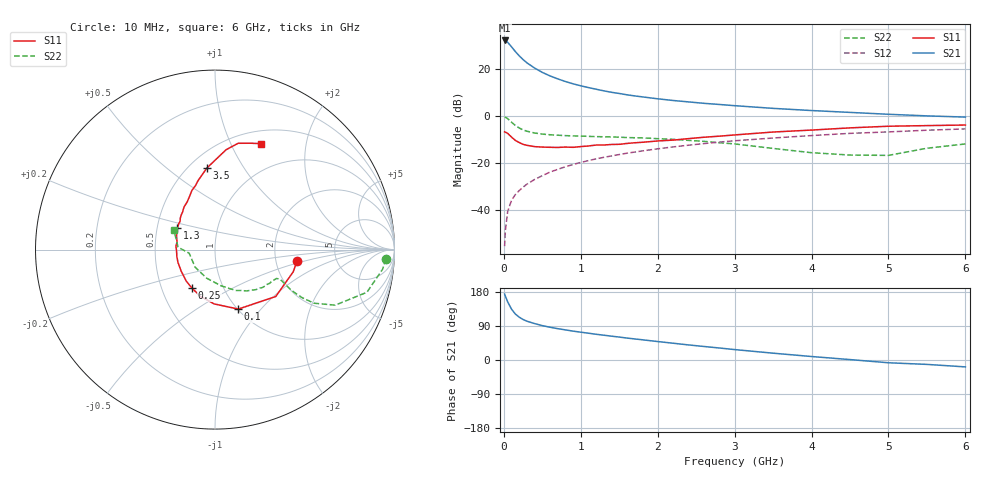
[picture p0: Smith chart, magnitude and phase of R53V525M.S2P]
! SIEMENS Small Signal Semiconductors
! BFR183
! Si NPN RF Bipolar Junction Transistor in SOT23
! VCE = 3.5 V  IC = 25 mA
! Common Emitter S-Parameters:  May  1996
# GHz  S  MA  R  50
!  f  S11  S21  S12  S22
! GHz  MAG  ANG  MAG  ANG  MAG  ANG  MAG  ANG
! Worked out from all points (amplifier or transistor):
!   36 points, 10 MHz to 6 GHz, reference 50 ohm
!   highest |S21| = 32.2 dB at 10 MHz (marker M1)
!   |S21| within 3 dB of that: start of sweep to 107.2 MHz
!   unconditionally stable (mu >= 1): 483.5 MHz to 2.364 GHz
!   at 250 MHz: K = 0.86, MSG = 27.2 dB, |S12| = -30.3 dB
!   at 1.4 GHz: K = 1.04, MAG = 12.3 dB, |S12| = -17.0 dB
!   at 6 GHz: K = 0.90, MSG = 2.5 dB, |S12| = -5.5 dB
!   S11 on the Smith chart (normalised r, x): 10 MHz: 2.63, -0.43; 100 MHz: 1.01, -0.76; 250 MHz: 0.71, -0.32; 1.3 GHz: 0.64, +0.16; 3.5 GHz: 0.61, +0.70; 6 GHz: 0.65, +1.31
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0.01  0.4613 -8.1  40.55 174.0  0.0017 85.6  0.9526 -3.1
0.02  0.4529 -15.9  39.98 168.4  0.0037 85.2  0.9402 -6.7
0.05  0.4276 -37.7  36.96 153.3  0.0093 78.9  0.879 -15.7
0.1  0.3559 -68.6  29.69 134.2  0.0161 71.8  0.7378 -24.8
0.15  0.3025 -91.0  23.49 121.2  0.0213 69.2  0.6283 -28.4
0.2  0.2722 -107.7  19.12 113.0  0.0259 69.5  0.5559 -28.9
0.25  0.2499 -121.0  15.88 106.9  0.0306 70.0  0.506 -28.4
0.3  0.2379 -132.2  13.55 102.4  0.0355 71.1  0.4745 -27.8
0.4  0.2232 -147.7  10.49 96.1  0.0447 72.0  0.4354 -26.2
0.5  0.2184 -160.6  8.476 90.7  0.0537 73.0  0.4125 -25.1
0.6  0.216 -169.6  7.146 86.5  0.0641 72.8  0.3994 -24.7
0.7  0.2144 -178.1  6.179 82.7  0.0733 73.0  0.3908 -24.7
0.8  0.2185 175.1  5.424 79.5  0.0831 72.1  0.3826 -25.0
0.9  0.2157 168.4  4.847 76.2  0.0931 71.5  0.3776 -25.3
1.1  0.2304 158.2  4.029 70.7  0.1125 70.3  0.3692 -27.5
1.3  0.2415 149.9  3.432 65.4  0.1322 68.6  0.3613 -29.6
1.7  0.2695 134.4  2.68 55.6  0.171 64.5  0.3449 -35.2
2.2  0.3075 120.3  2.141 44.3  0.22 59.0  0.3192 -44.3
3.5  0.4566 95.7  1.455 18.0  0.3405 42.4  0.2044 -80.5
4.5  0.5596 83.7  1.194 1.1  0.4274 29.6  0.1477 -138.7
5.5  0.6253 71.4  1.007 -11.6  0.4988 17.8  0.2062 176.2
6  0.6435 66.5  0.949 -18.2  0.5323 10.2  0.2546 154.3
